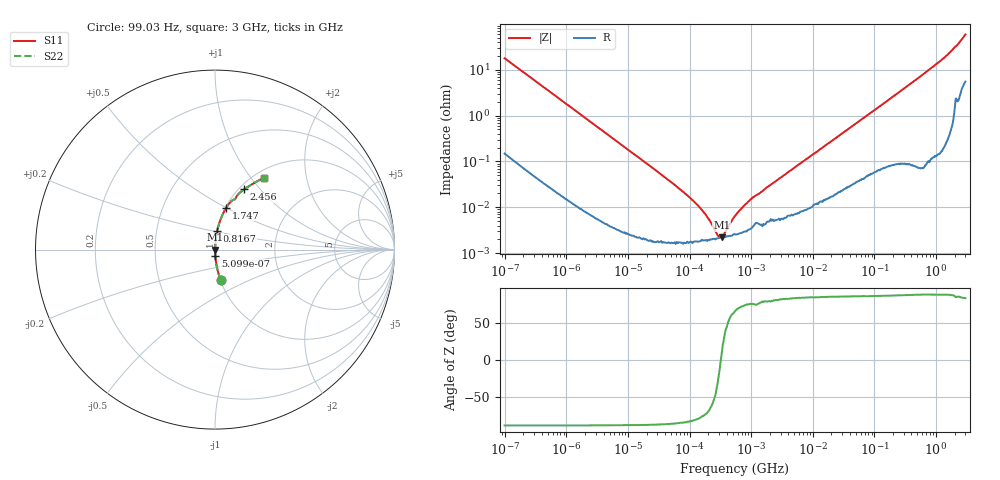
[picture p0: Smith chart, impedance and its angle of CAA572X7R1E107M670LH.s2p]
! S-Parameter Data Generated by TDK Corporation
! Copyright(C) 2023 TDK Corporation.
! All Rights Reserved.
! TDK P/N: CAA572X7R1E107M670LH (Multilayer Ceramic Chip Capacitor)
! Property: C=100uF
! Size(LxWxT): 6.25x5x6.7mm
! Model Type: s2p (Touchstone File Format Version 1.0)
! Frequency: DC=Yes Start=9.9035E-05MHz Stop=3000MHz 582points Log-sweep
! Model Generated on Mar. 24, 2023
! Port Assignments:
!  1 ---| |--- 2
! Applicable Conditions:
!  Temperature = 25 degC
!  DC Bias Voltage = 0 V
!  Small Signal Operation
! Terms and conditions regarding TDK Simulation Models
! (1)This simulation model is being provided solely for informational purposes. Please refer to the specifications of the products in terms of detailed characteristics of such products.
! (2)In no event shall TDK Corporation of any of its subsidiaries be liable for any loss or damage arising, directly or indirectly,
!  From any information contained in this simulation model, including, but not limited to loss or damages arising from any inaccuracies, omissions or errors in connection with such information.
! (3)Any and all copyrights on this simulation model are owned by TDK Corporation.
!  Duplication or redistribution of this simulation model without prior written permission from TDK Corporation is prohibited.
! (4)This simulation model is subject to any modification or change without any prior notice.
! (5)Neither TDK Corporation nor any of its subsidiaries shall make any warranty, express or implied,
!  Including but not limited to the correctness, implied warranties of merchantability and fitness for a particular purpose with respect to this simulation models.
! (6)The use of this simulation model shall be deemed to have consented to the terms and conditions hereof.
# Hz S MA R 50
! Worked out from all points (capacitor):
!   581 points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, 99.03 Hz to 3 GHz, reference 50 ohm
!   read as one part in series: C = 90.3 uF near 107.1 Hz
!   lowest |Z| = 2.2 mohm at 331.5 kHz (marker M1)
!   series resonance near 320.8 kHz, so ESL is about 2.7 nH
!   S11 on the Smith chart (normalised r, x): 99.03 Hz: 1.00, -0.35; 509.9 Hz: 1.00, -0.07; 816.7 MHz: 1.00, +0.21; 1.747 GHz: 1.01, +0.50; 2.456 GHz: 1.06, +0.82; 3 GHz: 1.11, +1.17
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99.035  0.1744 -79.5  0.9832 10.0  0.9832 10.0  0.1744 -79.5
207.851  0.08476 -84.7  0.9957 4.9  0.9957 4.9  0.08476 -84.7
509.913  0.0349 -87.5  0.9991 2.0  0.9991 2.0  0.0349 -87.5
1777.25  0.01009 -88.9  0.9999 0.6  0.9999 0.6  0.01009 -88.9
31893.81  0.0005633 -88.2  1 0.0  1 0.0  0.0005633 -88.2
72370.14  0.0002377 -85.9  1 0.0  1 0.0  0.0002377 -85.9
146075.1  9.86e-05 -79.4  1 0.0  1 0.0  9.86e-05 -79.4
157930.8  8.74e-05 -77.0  1 0.0  1 0.0  8.74e-05 -77.0
331458.5  2.201e-05 8.6  1 -0.0  1 -0.0  2.201e-05 8.6
550451.5  6.611e-05 67.3  1 -0.0  1 -0.0  6.611e-05 67.3
669030.6  8.968e-05 72.3  1 -0.0  1 -0.0  8.968e-05 72.3
752111.3  0.0001059 74.1  1 -0.0  1 -0.0  0.0001059 74.1
1068539  0.0001648 76.7  1 -0.0  1 -0.0  0.0001648 76.7
1404133  0.0002072 78.4  1 -0.0  1 -0.0  0.0002072 78.4
9878183  0.001405 85.7  0.9999 -0.1  0.9999 -0.1  0.001405 85.7
1.714156e8  0.0221 86.7  0.999 -1.3  0.999 -1.3  0.0221 86.7
4.135554e8  0.0526 86.1  0.9978 -3.0  0.9978 -3.0  0.0526 86.1
8.167498e8  0.1047 83.4  0.9934 -6.0  0.9934 -6.0  0.1047 83.4
1.243477e9  0.1625 80.1  0.9851 -9.4  0.9851 -9.4  0.1625 80.1
1.747494e9  0.242 74.9  0.9657 -14.0  0.9657 -14.0  0.242 74.9
2.455801e9  0.3724 64.3  0.9033 -21.8  0.9033 -21.8  0.3724 64.3
3e9  0.4862 55.7  0.8293 -29.0  0.8293 -29.0  0.4862 55.7
